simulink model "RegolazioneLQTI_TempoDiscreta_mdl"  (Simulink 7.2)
settings: Solver=ode45  StartTime=0.0  StopTime=10.0  RelTol=1e-3
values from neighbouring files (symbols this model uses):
  G = chol(Q)    [RegolazioneOttimaTempoInfinita_Integrale.m]    (also in RegolazioneOttimaTempoInfinita_uscita.m; RegolazioneOttimaTempoInfinita_uscita_osservatore.m; RegolazioneOttimaTempoInfinita.m)
  Ts = 0.01    [RegolazioneOttimaTempoInfinita_TempoDiscreto.m]    (also in ControlloOttimoTempoInfinito_TempoDiscreto.m)
  X0 = [2;-3]    [RegolazioneOttimaTempoInfinita_Integrale.m]    (also in RegolazioneOttimaTempoInfinita_TempoDiscreto.m; RegolazioneOttimaTempoInfinita_uscita.m; RegolazioneOttimaTempoInfinita_uscita_osservatore.m; RegolazioneOttimaTempoInfinita.m)
undefined symbols (not defined in the file or in its folder): F, Kd

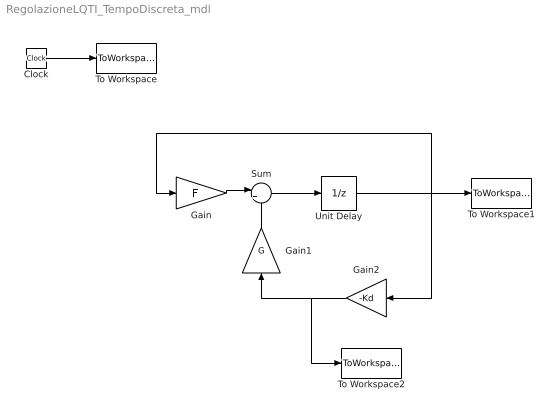
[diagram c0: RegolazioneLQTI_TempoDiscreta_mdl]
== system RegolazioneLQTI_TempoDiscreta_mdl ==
  Clock : Clock
  Gain : Gain  Gain=F  Multiplication=Matrix(K*u)  ParameterDataType=sfix(16)  ParameterScaling=2^0  OutDataType=sfix(16)  OutScaling=2^0
  Gain1 : Gain  Orientation=up  Gain=G  Multiplication=Matrix(K*u)  ParameterDataType=sfix(16)  ParameterScaling=2^0  OutDataType=sfix(16)  OutScaling=2^0
  Gain2 : Gain  Orientation=left  Gain=-Kd  Multiplication=Matrix(K*u)  ParameterDataType=sfix(16)  ParameterScaling=2^0  OutDataType=sfix(16)  OutScaling=2^0
  Sum : Sum  Inputs=|++  OutDataType=sfix(16)  OutScaling=2^0
  To Workspace : ToWorkspace  VariableName=time  SampleTime=-1  SaveFormat=Array
  To Workspace1 : ToWorkspace  VariableName=X  SampleTime=-1  SaveFormat=Array
  To Workspace2 : ToWorkspace  VariableName=u  SampleTime=-1  SaveFormat=Array
  Unit Delay : UnitDelay  X0=X0  SampleTime=Ts
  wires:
  Gain/1 -> Sum/1
  Unit Delay/1 -> Gain/1, Gain2/1, To Workspace1/1
  Gain1/1 -> Sum/2
  Gain2/1 -> Gain1/1, To Workspace2/1
  Sum/1 -> Unit Delay/1
  Clock/1 -> To Workspace/1
